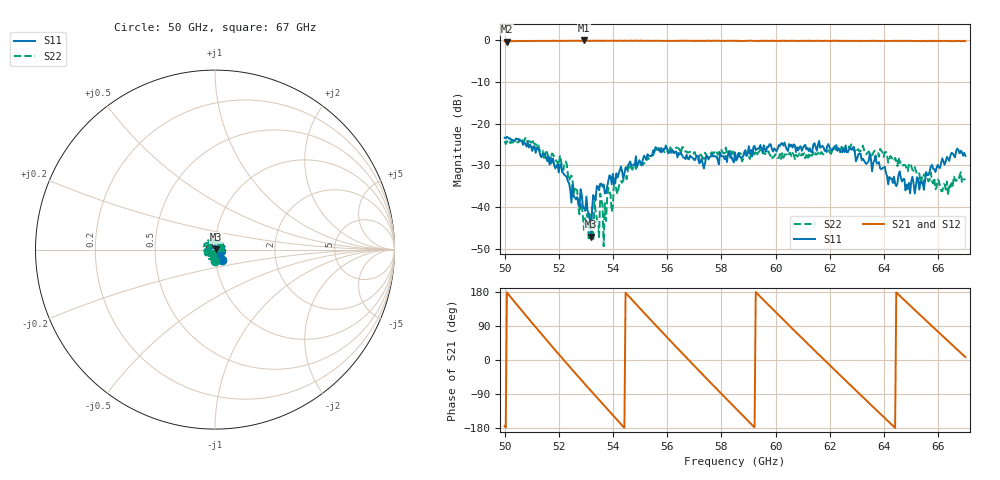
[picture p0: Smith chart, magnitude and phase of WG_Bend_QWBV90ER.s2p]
!Agilent Technologies,E8361A,US42410132,A.06.03.05
!Agilent E8361A: A.06.03.05
!Date: Friday, July 11, 2008 16:24:56
!Correction: S11(Full 2 Port(1,2)) S21(Full 2 Port(1,2)) S12(Full 2 Port(1,2)) S22(Full 2 Port(1,2))
!S2P File: Measurements: S11, S21, S12, S22:
# Hz S  MA  R 50
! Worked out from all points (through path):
!   401 points, 50 GHz to 67 GHz, reference 50 ohm
!   highest |S21| = -0.07 dB at 52.93 GHz (marker M1); lowest = -0.3 dB at 50.09 GHz (marker M2)
!   lowest |S11| = -47.1 dB at 53.19 GHz (marker M3), VSWR 1.01, Z = 50.4 + j0.148 ohm
!   |S11| at or under -10 dB: start of sweep to end of sweep
!   |S22| runs from -49.4 to -23.4 dB; largest |S21 - S12| = 0.019
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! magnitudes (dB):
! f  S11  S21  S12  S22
! 50 GHz  -23.4  -0.3  -0.2  -24.2
! 50.09 GHz  -23.2  -0.3  -0.2  -24.2
! 50.98 GHz  -25.5  -0.2  -0.2  -24.6
! 52.21 GHz  -32.3  -0.1  -0.2  -29.5
! 52.85 GHz  -37.1  -0.1  -0.1  -39.5
! 52.93 GHz  -40.2  -0.1  -0.1  -45.5
! 53.19 GHz  -47.1  -0.1  -0.1  -43.9
! 53.48 GHz  -36.0  -0.2  -0.1  -47.2
! 53.7 GHz  -36.8  -0.1  -0.2  -39.1
! 53.78 GHz  -35.1  -0.1  -0.2  -37.8
! 54.63 GHz  -29.1  -0.2  -0.1  -29.7
! 55.7 GHz  -26.3  -0.2  -0.1  -25.8
! 57.27 GHz  -28.4  -0.2  -0.1  -27.7
! 58.5 GHz  -26.9  -0.2  -0.1  -27.5
! 60.24 GHz  -24.7  -0.1  -0.1  -27.1
! 61.35 GHz  -26.9  -0.2  -0.1  -27.7
! 62.79 GHz  -26.3  -0.2  -0.1  -25.0
! 64.19 GHz  -32.8  -0.2  -0.2  -28.5
! 65.39 GHz  -34.2  -0.2  -0.2  -32.8
! 65.77 GHz  -29.9  -0.3  -0.2  -33.8
! 66.19 GHz  -29.2  -0.2  -0.2  -34.5
! 67 GHz  -27.7  -0.3  -0.3  -33.3
